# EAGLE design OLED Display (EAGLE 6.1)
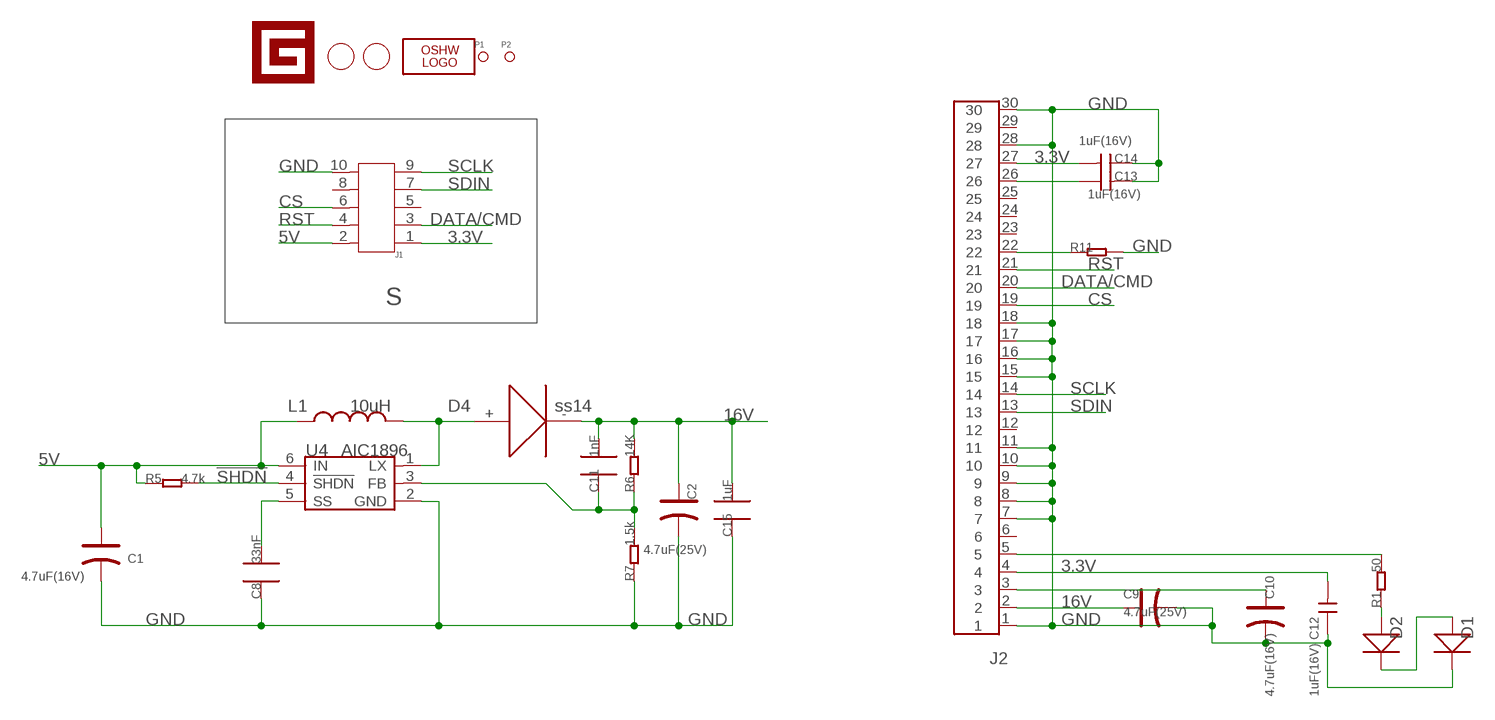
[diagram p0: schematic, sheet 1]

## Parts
C1  4.7uF(16V)  CAP_AVX_A  [AVX-A]
C2  4.7uF(25V)  CAP_AVX_C  [AVX-C]
C8  33nF  C0603_S  [0603_S]
C9  4.7uF(25V)  CAP_AVX_C  [AVX-C]
C10  4.7uF(16V)  CAP_AVX_A  [AVX-A]
C11  1nF  C0603_S  [0603_S]
C12  1uF(16V)  C-0603  [0603]
C13  1uF(16V)  C-0603  [0603]
C14  1uF(16V)  C-0603  [0603]
C15  1uF  C0805_S  [0805_S]
D1  D-0805  [SOD323]
D2  D-0805  [SOD323]
D4  ss14  DIODE2010  [DIODE_2010]
J1  HEADER-SHF-105-01-L-D-SM  [SHF-105-01-L-D-SM]
J2  FPC-SOCKET-0.5-30P  [30P-0.5-90D-18.4X5.0]
L1  10uH  INDUCTOR_6062  [6062]
LOGO1  LOGO-OSHW-FILLX0150-NT  [OSHW_FILLX150_NOTEXT]
P1  PAD-MARK  [ROUND-MARK-0.635]
P2  PAD-MARK  [ROUND-MARK-0.635]
R1  50  R-0603  [0603]
R5  4.7k  R0603_S  [0603_S]
R6  14K  R0603_S  [0603_S]
R7  1.5k  R0603_S  [0603_S]
R11  R-0603  [0603]
U4  AIC1896  [SOT23-6]
U$1  LOGO-GADGETEER-NORMAL  [GADGETEER-SILK]
U$2  PAD-HOLE'3.2/7.0'  [HOLE-D-3.2/7.0]
U$3  PAD-HOLE'3.2/7.0'  [HOLE-D-3.2/7.0]

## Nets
3.3V: C12.2 C14.2 J1.1 J2.4 J2.27
5V: C1.+ J1.2 L1.1 R5.1 U4.6(IN)
16V: C2.+ C9.+ C11.2 C15.2 D4.- J2.2 R6.2
!SHDN: R5.2 U4.4(!SHDN)
CS: J1.6 J2.19
DATA/CMD: J1.3 J2.20
GND: C1.- C2.- C8.1 C9.- C10.- C12.1 C13.2 C14.1 C15.1 D1.- J1.10 J2.1 J2.7 J2.8 J2.9 J2.10 J2.11 J2.15 J2.16 J2.17 J2.18 J2.28 J2.30 R7.1 R11.2 U4.2(GND)
N$1: C13.1 J2.26
N$2: C10.+ J2.3
N$3: D1.+ D2.-
N$8: C8.2 U4.5(SS)
N$9: D4.+ L1.2 U4.1(LX)
N$10: J2.5 R1.2
N$11: C11.1 R6.1 R7.2 U4.3(FB)
N$12: D2.+ R1.1
N$13: J2.22 R11.1
RST: J1.4 J2.21
SCLK: J1.9 J2.14
SDIN: J1.7 J2.13
Unconnected: J1.5 J1.8 J2.6 J2.12 J2.23 J2.24 J2.25 J2.29

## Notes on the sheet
- S

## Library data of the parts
C1 C2 C9 C10 = Discrete:CAP*: Electrolytic Capacitors,Tantalum Capacitors and Super Capacitors
C8 C11 = CPT_SMD:C0603
C12-C14 = Discrete:C*: Ceramic Capacitors
C15 = CPT_SMD:C0805
D1 D2 = Discrete:D*
D4 = CPT_SMD:DIODE
J1 = Connector:HEADER-SHF-105-01-L-D-SM
J2 = Connector:FPC-SOCKET-0.5-30P
L1 = CPT_SMD:INDUCTOR
LOGO1 = Logo:LOGO-OSHW-FILL
P1 P2 = Discreter:PAD-MARK
R1 R11 = Discrete:R*
R5-R7 = CPT_SMD:R0603
U4 = ICs_v54:AIC1896
U$1 = Logo:LOGO-GADGETEER
U$2 U$3 = Discreter:PAD-HOLE

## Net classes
0 default: width 0.152 mm, drill 0.305 mm, clearance 0.152 mm

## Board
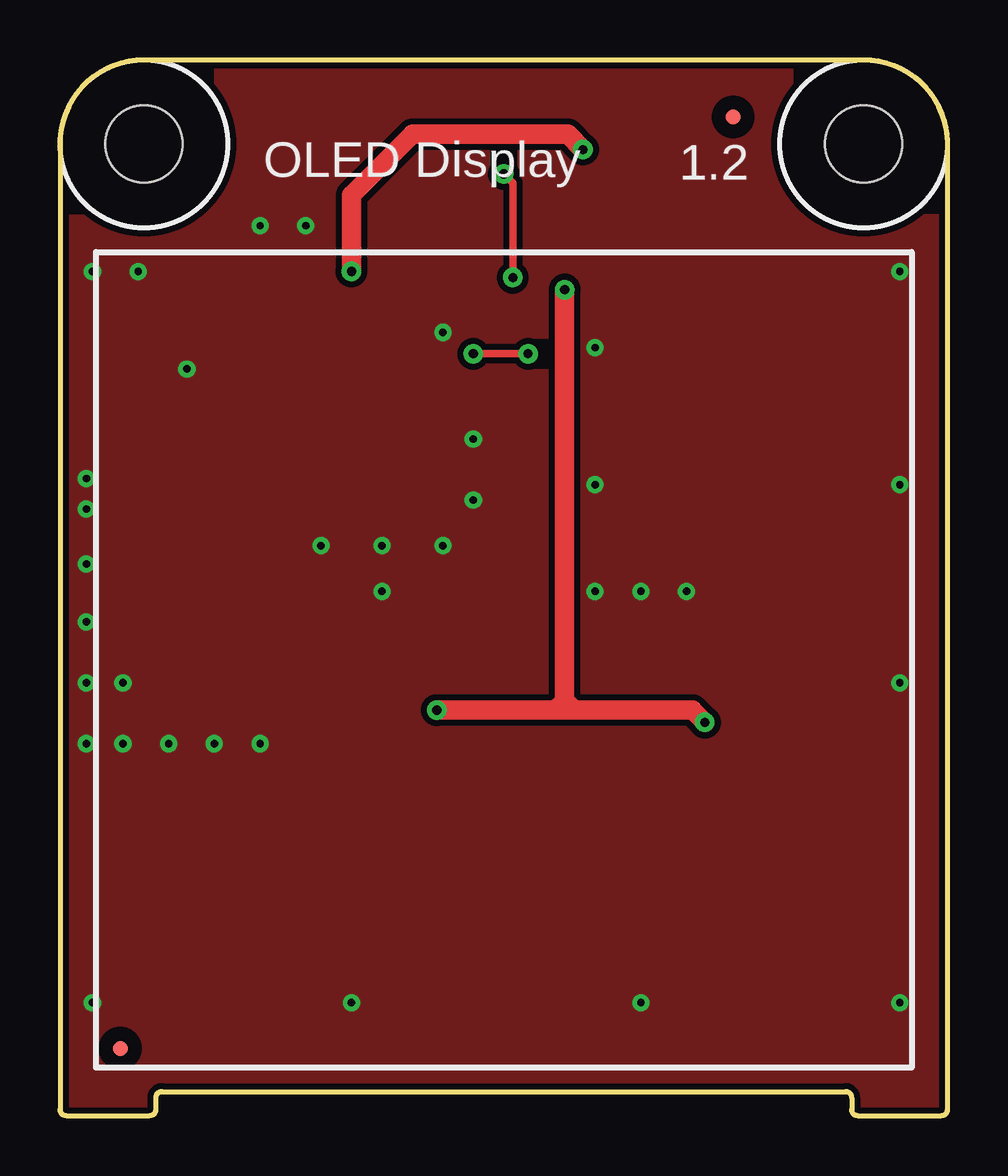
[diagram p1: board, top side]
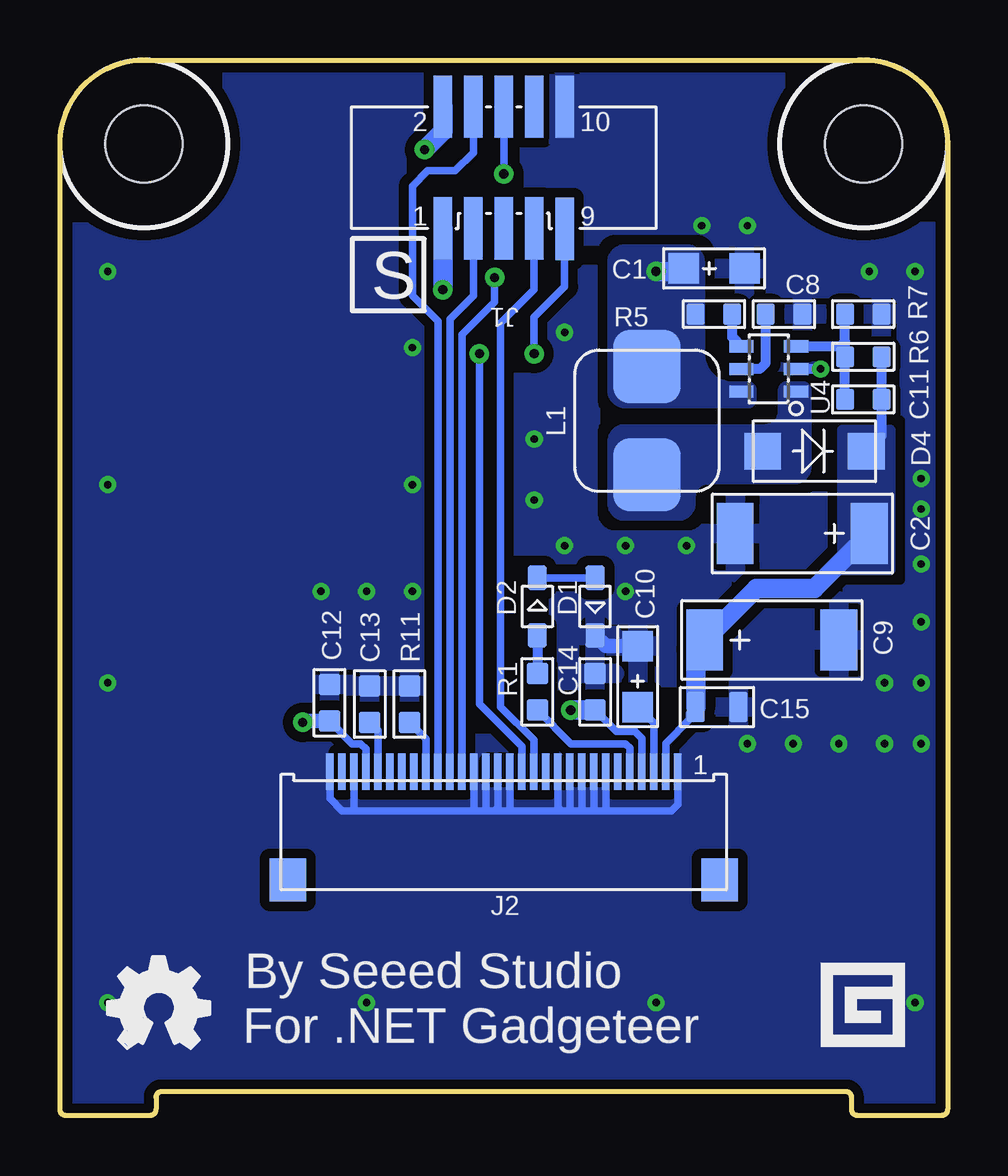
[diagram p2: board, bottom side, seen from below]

Size 37 x 44 mm. Coordinates in mm from the lower left corner, seen from the top.
Outline: 37,40.5 arc90 33.5,44 3.5,44 arc90 0,40.5 0,0.25 arc90 0.25,0 3.75,0 arc90 4,0.25 4,0.75 arc-90 4.25,1 32.75,1 arc-90 33,0.75 33,0.25 arc90 33.25,0 36.75,0 arc90 37,0.25 37,40.5
Copper layers (1*16): Top 0.035mm / dielectric 1.5mm / Bottom 0.035mm
Design rules: minimum track width 10mil, minimum drill 12mil, track to track 6mil, track to pad 6mil, pad to pad 6mil, via to via 6mil, smd to smd 0mil, copper to edge 10mil, drill to drill 8mil, minimum pad ring 10mil, minimum via ring 8mil, stop-mask expansion 4mil, vias tented up to drill 100mil, thermal gap 10mil
bRestrict: area 14.4,14.1 to 14.6,14.7; area 14.9,14.1 to 15.1,14.7; area 15.3,14.1 to 15.5,14.7; area 19,14.1 to 19.1,14.7; area 18.5,14.1 to 18.6,14.7; area 16,14 to 16.1,14.6

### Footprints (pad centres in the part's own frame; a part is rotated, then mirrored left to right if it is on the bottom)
AVX-A = smd 1.27 x 1.27: + -1.27,0; - 1.27,0
AVX-C = smd 1.524 x 2.54: + -2.794,0; - 2.794,0
0603_S = smd 0.762 x 0.889: 1 -0.762,0; 2 0.762,0
0603 = smd 0.889 x 0.889: 1 -0.762,0; 2 0.762,0
0805_S = smd 0.762 x 1.27: 1 -0.889,0; 2 0.889,0
SOD323 = smd 1 x 0.8: + -1.2,0; - 1.2,0
DIODE_2010 = smd 1.524 x 1.524: + 0,-2.159; - 0,2.159
SHF-105-01-L-D-SM = smd 0.762 x 2.6: 1 -2.54,-2.54; 2 -2.54,2.54; 3 -1.27,-2.54; 4 -1.27,2.54; 5 0,-2.54; 6 0,2.54; 7 1.27,-2.54; 8 1.27,2.54; 9 2.54,-2.546; 10 2.54,2.54
30P-0.5-90D-18.4X5.0 = smd 0.305 x 1.524: 1 7.25,2; 2 6.75,2; 3 6.25,2; 4 5.75,2; 5 5.25,2; 6 4.75,2; 7 4.25,2; 8 3.75,2; 9 3.25,2; 10 2.75,2; 11 2.25,2; 12 1.75,2; 13 1.25,2; 14 0.75,2; 15 0.25,2; 16 -0.25,2; 17 -0.75,2; 18 -1.25,2; 19 -1.75,2; 20 -2.25,2; 21 -2.75,2; 22 -3.25,2; 23 -3.75,2; 24 -4.25,2; 25 -4.75,2; 26 -5.25,2; 27 -5.75,2; 28 -6.25,2; 29 -6.75,2; 30 -7.25,2 | smd 1.524 x 1.778: P$1 -9,-2.5; P$2 9,-2.5
6062 = smd 2.794 x 3.048: 1 0,2.254; 2 0,-2.254
ROUND-MARK-0.635 = smd 0.635 x 0.635: P$1 0,0
SOT23-6 = smd 0.508 x 1.016: 1 -0.94,-1.143; 2 0,-1.143; 3 0.94,-1.143; 4 0.94,1.143; 5 0,1.143; 6 -0.94,1.143
HOLE-D-3.2/7.0 = hole 3.2: 0,0

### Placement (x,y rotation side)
C1  9.74,35.31 0 bottom
C2  6.05,24.26 180 bottom
C8  6.82,33.41 180 bottom
C9  7.32,19.82 0 bottom
C10  12.91,18.29 90 bottom
C11  3.51,29.85 0 bottom
C12  25.76,17.2 270 bottom
C13  24.09,17.15 90 bottom
C14  14.69,17.66 270 bottom
C15  9.61,17.02 180 bottom
D1  14.69,21.21 270 bottom
D2  17.1,21.21 90 bottom
D4  5.55,27.69 270 bottom
J1  18.5,39.51 0 bottom
J2  18.5,12.32 0 bottom
L1  12.53,28.96 0 bottom
LOGO1  35.01,2.8 0 bottom
P1  2.51,2.8 180 top
P2  28.06,41.62 0 top
R1  17.1,17.66 270 bottom
R5  9.74,33.41 0 bottom
R6  3.51,31.63 0 bottom
R7  3.51,33.41 180 bottom
R11  22.44,17.15 90 bottom
U4  7.45,31.12 90 bottom
U$1  3.12,5.05 0 bottom
U$2  33.5,40.5 0 top
U$3  3.5,40.5 0 top

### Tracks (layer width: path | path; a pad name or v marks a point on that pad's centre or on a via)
3.3V  (via drill 0.38 pad 0.81)
  Top 0.813: 21.04,16.9 v15.71,16.9 | 21.04,17.28 21.04,16.9 | 21.04,17.28 21.29,17.02 20.79,17.02 21.04,17.28 | 21.04,17.28 v21.04,34.42 | 21.04,16.9 26.37,16.9 v26.88,16.39
  Bottom 0.305: C14.2 13.8,16.01 13.04,16.01 12.75,15.72 J2.4 | J2.27 24.25,15.28 24.47,15.5 24.82,15.5 C12.2
  Bottom 0.61: C12.2 26.83,16.44 v26.88,16.39
  Bottom 0.813: v21.04,34.42 J1.1 | v15.71,16.9 C14.2
5V  (via drill 0.38 pad 0.81)
  Top 0.813: v12.15,35.19 12.15,38.36 14.69,40.9 21.17,40.9 v21.8,40.27
  Bottom 0.813: J1.2 21.04,41.03 v21.8,40.27 | v12.15,35.19 11.13,35.19 C1.+
  pour Bottom (isolate 0.254, no thermals): 13.42,29.6 arc90 14.05,30.23 14.05,35.57 arc90 13.42,36.2 10.88,36.2 arc90 10.24,35.57 10.24,31.76 arc-90 8.97,30.49 8.34,30.49 arc90 8.09,30.23 8.09,29.85 arc90 8.34,29.6
16V
  Bottom 0.305: 10.5,16.9 C15.2 10.75,16.77 10.75,16.52 11.75,15.52 J2.2
  Bottom 0.406: R6.2 C11.2 2.75,28.33 D4.- | C2.+ 3.39,24.39
  Bottom 0.813: C2.+ 5.55,21.98 7.96,21.98 C9.+ 10.5,19.44 C15.2
  pour Bottom (isolate 0.254, no thermals): 4.4,22.74 2.37,22.74 2.37,28.58 4.4,28.58
!SHDN
  Bottom 0.406: R5.2 8.97,32.44 U4.4
CS  (via drill 0.38 pad 0.81)
  Top 0.305: v18.88,34.93 18.88,38.87 v18.5,39.25
  Bottom 0.305: v18.88,34.93 18.88,33.91 20.25,32.55 20.25,31.6 J2.19 | v18.5,39.25 J1.6
DATA/CMD
  Bottom 0.305: J1.3 19.77,34.17 20.75,33.19 20.75,31.21 J2.20
GND  (via drill 0.3 pad 0.64)
  Bottom 0.305: J2.7 14.25,12.77 14.18,12.71 | 14.18,12.71 11.52,12.71 11.25,12.97 J2.1 | 14.18,12.71 14.82,12.71 | 14.82,12.71 15.2,12.71 | 15.2,12.71 15.71,12.71 | 15.71,12.71 16.09,12.71 | 16.09,12.71 18.25,12.71 | 18.25,12.71 18.88,12.71 | 18.88,12.71 19.26,12.71 | 19.26,12.71 19.64,12.71 | 19.64,12.71 24.72,12.71 | 24.72,12.71 25.23,12.71 25.75,13.22 J2.30 | J2.28 24.75,12.73 24.72,12.71 | J2.18 19.75,12.81 19.64,12.71 | J2.17 19.25,12.72 19.26,12.71 | J2.16 18.75,12.84 18.88,12.71 | J2.15 18.25,12.71 | J2.11 16.25,12.87 16.09,12.71 | J2.10 15.75,12.75 15.71,12.71 | J2.9 15.25,12.76 15.2,12.71 | J2.8 14.75,12.77 14.82,12.71
  Bottom 0.406: v5.29,31.12 U4.2
  Bottom 0.61: C10.- 14.24,19.56 D1.-
  other vias: 3.26,35.19 1.1,18.04 1.1,20.58 24.21,4.71 35.01,4.71 10.88,23.76 13.42,21.85 15.96,23.76 13.42,23.76 1.1,22.99 1.1,25.28 1.1,26.55 17.23,28.2 17.23,25.66 15.96,32.64 2.62,18.04 2.62,15.5 1.1,15.5 4.53,15.5 6.44,15.5 8.34,15.5 1.36,35.19 8.34,37.09 10.24,37.09 12.15,4.71 1.36,4.71 35.01,18.04 35.01,26.3 35.01,35.19 22.31,21.85 24.21,21.85 26.12,21.85 22.31,26.3 22.31,32.01
  pour Bottom (isolate 0.406, rank 5): -1.5,45.5 38.5,45.5 38.5,-2 -1.5,-2
  pour Top (isolate 0.254): -1.5,45.5 38.5,45.5 38.5,-2 -1.5,-2
  pour Bottom (isolate 0.254, no thermals): 16.59,40.61 14.31,40.61 14.31,43.28 16.59,43.28
N$1
  Bottom 0.305: 23.83,16.14 C13.1 23.75,16.05 J2.26
N$2
  Bottom 0.305: C10.+ 12.25,16.36 12.25,16.16 J2.3
N$3
  Bottom 0.305: D1.+ D2.-
N$8
  Bottom 0.406: U4.5 7.83,31.12 7.58,31.38 C8.2
N$9
  pour Bottom (isolate 0.254, no thermals): 5.8,27.06 arc90 6.44,26.42 9.99,26.42 arc-90 10.63,25.79 10.63,25.53 arc90 11.26,24.9 13.42,24.9 arc90 14.05,25.53 14.05,28.07 arc90 13.42,28.71 7.58,28.71 arc-90 6.94,29.34 6.94,30.23 arc90 6.69,30.49 6.05,30.49 arc90 5.8,30.23
N$10
  Bottom 0.305: J2.5 13.25,15.33 13.42,15.5 15.71,15.5 R1.2
N$11
  Bottom 0.406: C11.1 R6.1 4.28,32.14 | 4.28,32.14 4.28,32.26 | 4.28,32.26 R7.2 | 4.48,32.06 4.35,32.06 4.28,32.14 | 4.48,32.06 U4.3 | 4.28,32.26 4.48,32.06
N$12
  Bottom 0.406: D2.+ R1.1
N$13
  Bottom 0.305: J2.22 21.75,15.7 R11.1
RST
  Bottom 0.305: J1.4 19.77,40.14 20.53,39.38 21.68,39.38 22.31,38.74 22.31,34.17 21.25,33.11 J2.21
SCLK  (via drill 0.38 pad 0.81)
  Top 0.305: v19.52,31.76 v17.23,31.76
  Bottom 0.305: v19.52,31.76 19.52,17.15 17.75,15.38 J2.14 | J1.9 15.96,34.55 17.23,33.28 v17.23,31.76
SDIN
  Bottom 0.305: J1.7 17.23,34.42 18.63,33.03 18.63,17.02 17.25,15.65 J2.13

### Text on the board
tPlace: 1.2 | OLED Display
bPlace: S | 1 | By Seeed Studio | For .NET Gadgeteer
